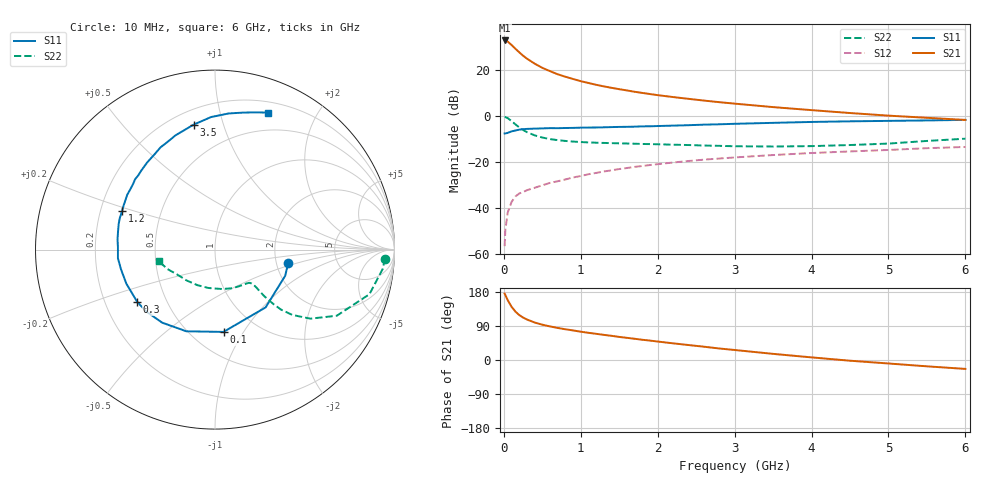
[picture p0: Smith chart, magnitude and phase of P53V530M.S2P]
! SIEMENS Small Signal Semiconductors
! BFP183
! Si NPN RF Bipolar Junction Transistor in SOT143
! VCE = 3.5 V  IC = 30 mA
! Common Emitter S-Parameters:  March  1996
# GHz  S  MA  R  50
!  f  S11  S21  S12  S22
! GHz  MAG  ANG  MAG  ANG  MAG  ANG  MAG  ANG
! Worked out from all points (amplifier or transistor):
!   36 points, 10 MHz to 6 GHz, reference 50 ohm
!   highest |S21| = 32.7 dB at 10 MHz (marker M1)
!   |S21| within 3 dB of that: start of sweep to 132.2 MHz
!   unconditionally stable (mu >= 1): 646.1 MHz to 5.594 GHz
!   at 250 MHz: K = 0.60, MSG = 29.6 dB, |S12| = -33.0 dB
!   at 1.4 GHz: K = 1.17, MAG = 15.4 dB, |S12| = -23.6 dB
!   at 6 GHz: K = 0.95, MSG = 5.9 dB, |S12| = -13.5 dB
!   S11 on the Smith chart (normalised r, x): 10 MHz: 2.33, -0.41; 100 MHz: 0.70, -0.82; 300 MHz: 0.34, -0.27; 1.2 GHz: 0.29, +0.18; 3.5 GHz: 0.29, +0.80; 6 GHz: 0.31, +1.42
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0.01  0.4147 -10.0  43.13 175.3  0.0015 81.9  0.9488 -3.0
0.02  0.4174 -20.5  42.93 171.1  0.0034 82.7  0.9404 -6.6
0.05  0.428 -48.8  40.79 158.0  0.008 77.3  0.8958 -16.1
0.1  0.461 -84.1  34.4 140.6  0.0136 62.3  0.7722 -28.5
0.15  0.4823 -109.3  28.58 127.8  0.0179 56.1  0.6561 -35.9
0.2  0.5022 -125.8  23.87 118.7  0.0208 52.8  0.5639 -40.2
0.25  0.5151 -137.8  20.15 112.0  0.0223 51.8  0.4957 -42.3
0.3  0.5222 -146.2  17.44 106.9  0.0245 51.4  0.4446 -43.0
0.4  0.5292 -159.1  13.58 99.0  0.0276 52.5  0.3788 -43.4
0.5  0.5353 -168.3  11 93.2  0.0313 52.8  0.3396 -43.0
0.6  0.5429 -174.9  9.323 88.6  0.0353 55.0  0.314 -42.5
0.7  0.541 178.6  7.975 84.6  0.0383 56.3  0.298 -42.4
0.8  0.5461 174.0  7.056 81.1  0.0419 56.4  0.2864 -42.4
1.1  0.5589 161.6  5.166 71.7  0.0544 57.4  0.266 -44.1
1.2  0.5603 157.5  4.721 69.1  0.0581 57.0  0.2624 -45.2
1.7  0.5842 141.5  3.332 56.0  0.0784 55.0  0.2494 -52.8
2.2  0.6154 127.8  2.559 44.0  0.0976 51.0  0.2374 -63.0
2.8  0.6572 113.3  1.984 30.4  0.119 45.3  0.2243 -78.5
3.5  0.7063 99.7  1.549 16.2  0.1417 39.0  0.2169 -99.7
4.5  0.7622 84.3  1.153 -1.9  0.1697 29.7  0.2335 -132.7
5.5  0.7967 73.7  0.909 -16.7  0.1995 21.5  0.2863 -157.8
6  0.8191 68.7  0.817 -23.5  0.212 16.8  0.3204 -168.5
